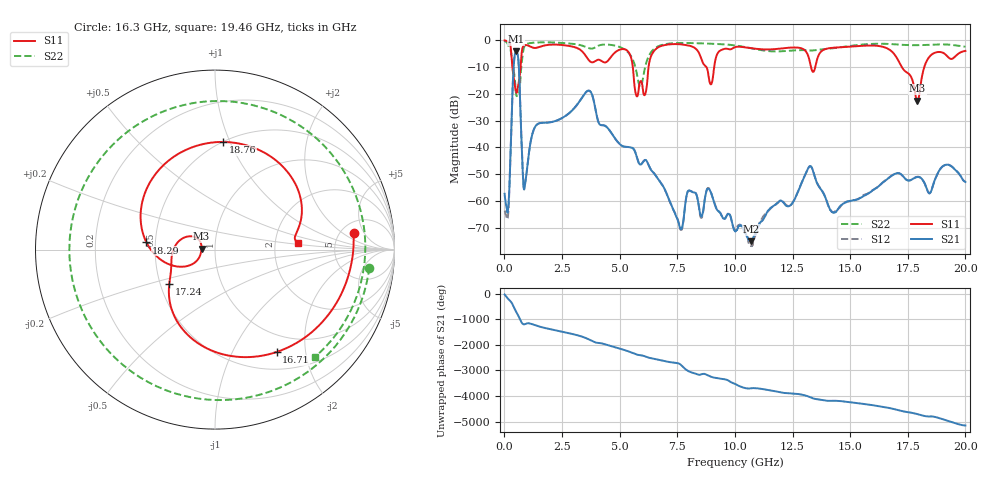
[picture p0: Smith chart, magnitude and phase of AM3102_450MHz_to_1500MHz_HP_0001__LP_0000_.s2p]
!Agilent Technologies,E8364B,MY43040894,A.07.50.67
!Agilent E8364B: A.07.50.67
!Date: Thursday, January 11, 2018 05:19:38
!Correction: S11(Full 2 Port(1,2))
!S21(Full 2 Port(1,2))
!S12(Full 2 Port(1,2))
!S22(Full 2 Port(1,2))
!S2P File: Measurements: S11, S21, S12, S22:
# Hz S  dB  R 50
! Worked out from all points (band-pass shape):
!   1601 points, 10 MHz to 20 GHz, reference 50 ohm
!   highest |S21| = -4.15 dB at 509.8 MHz (marker M1); lowest = -75.1 dB at 10.7 GHz (marker M2)
!   |S21| within 3 dB of the highest: 427.7 MHz to 605 MHz (177.3 MHz wide, 34.3 % of centre)
!   lowest |S11| = -22.5 dB at 17.91 GHz (marker M3), VSWR 1.16, Z = 43 + j0.468 ohm
!   |S11| at or under -10 dB: 347.4 MHz to 702.5 MHz (355.1 MHz wide, 67.6 % of centre); 5.573 GHz to 6.254 GHz (681.7 MHz wide, 11.5 % of centre); 17.24 GHz to 18.22 GHz (973 MHz wide, 5.49 % of centre)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
!   |S22| runs from -20.9 to -0.3 dB; largest |S21 - S12| = 0.0017
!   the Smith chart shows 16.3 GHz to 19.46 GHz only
!   S11 on the Smith chart (normalised r, x): 16.3 GHz: 6.59, +2.99; 16.71 GHz: 0.73, -1.51; 17.24 GHz: 0.56, -0.24; 18.29 GHz: 0.45, +0.04; 18.76 GHz: 0.50, +0.95; 19.46 GHz: 2.69, +0.24
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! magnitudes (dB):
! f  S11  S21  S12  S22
! 10 MHz  0.0  -57.3  -63.6  -0.3
! 172.4 MHz  -0.6  -62.3  -64.1  -2.0
! 509.8 MHz  -18.6  -4.2  -4.2  -20.2
! 884.6 MHz  -1.8  -54.5  -54.3  -2.1
! 1.359 GHz  -2.8  -32.0  -32.0  -0.8
! 3.346 GHz  -3.9  -21.7  -21.7  -1.9
! 5.307 GHz  -3.7  -39.8  -39.8  -4.0
! 5.745 GHz  -20.9  -43.6  -43.6  -12.3
! 6.682 GHz  -2.6  -51.9  -52.0  -2.2
! 10.01 GHz  -2.5  -71.1  -70.8  -1.9
! 10.7 GHz  -2.9  -75.1  -76.7  -2.9
! 13.34 GHz  -11.2  -47.6  -47.6  -3.8
! 14.28 GHz  -2.8  -64.4  -64.1  -2.9
! 16.3 GHz  -2.2  -54.0  -54.0  -1.3
! 16.68 GHz  -3.3  -51.4  -51.3  -1.3
! 16.71 GHz  -3.5  -51.1  -51.1  -1.4
! 17.24 GHz  -9.9  -50.3  -50.3  -1.7
! 17.91 GHz  -22.5  -51.0  -50.9  -1.8
! 18.29 GHz  -8.3  -54.6  -54.7  -1.7
! 18.76 GHz  -4.4  -50.3  -50.4  -1.5
! 19.46 GHz  -6.7  -47.5  -47.5  -1.8
! 20 GHz  -4.0  -52.9  -52.8  -2.4
